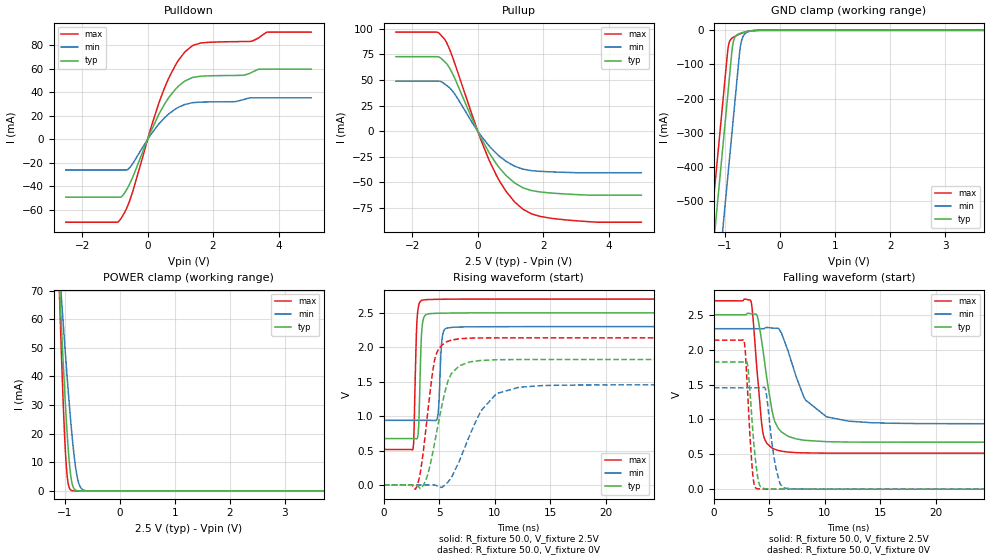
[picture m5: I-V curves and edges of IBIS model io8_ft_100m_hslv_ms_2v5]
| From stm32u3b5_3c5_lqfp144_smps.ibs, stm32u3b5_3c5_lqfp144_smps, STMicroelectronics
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[Model]   io8_ft_100m_hslv_ms_2v5
Model_type I/O
Polarity   Non-Inverting
Enable   Active-Low
| CAP_THRESHOLD on pad IOFT is "UDTCAPC" :
| Rising=30.0% of vddiom   Falling=70.0% of vddiom
| C_comp min and max val. don't necessarily correlate with the min and max pvt
| but are the smallest and greatest pad capacitance found.
| var   typ   min   max
C_comp   3.68195pF  3.67098pF  3.72549pF
|C_comp_pullup   2.08701pF  2.19344pF  2.32528pF
|C_comp_pulldown   1.59494pF  1.47754pF  1.40021pF
Vinl = 1.15V
Vinh = 1.35V
Vmeas = 1.25V   | Reference voltage for timing measurements
Cref  = 50.0pF   | Timing specification test load capacitance value
Rref  = 1.0MOhm   | Timing specification test load resistance value
Vref  = 1.375V   | Timing specification test load voltage
[Model Spec]
| TIME_THRESHOLD on pin ZIV11 is "CMOS" :
| Rising=50.0% of vdd   Falling=50.0% of vdd
Vinl 981.50000mV 911.50000mV 1.04650V
Vinh 1.42350V 1.31650V 1.50350V
| variable   typ   min   max
[Temperature Range] 25.0 130.0 -40.0
| variable   typ   min   max
[Voltage Range] 2.5V 2.3V 2.7V
| variable   typ   min   max
[POWER Clamp Reference] 2.5V 2.3V 2.7V
| variable   typ   min   max
[GND Clamp Reference] 0V 0V 0V
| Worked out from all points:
|   slope of the pulldown table from 0 to 0.375 V, typ, clamps not added: 16.4 ohm
|   slope of the pullup table from 0 to 0.375 V, typ, clamps not added: 16.7 ohm
|   GND clamp passes 1 mA (typ) near -0.50 V on its own axis
|   POWER clamp passes 1 mA (typ) near -0.83 V on its own axis
|   rising waveform, R_fixture 50.0, V_fixture 2.5V: 20-80 % time 200ps typ, 221ps min, 204ps max; typ from 0.673 V to 2.5 V
|   falling waveform, R_fixture 50.0, V_fixture 2.5V: 20-80 % time 1.06ns typ, 2.21ns min, 676ps max; typ from 2.5 V to 0.673 V
|   rising waveform, R_fixture 50.0, V_fixture 0V: 20-80 % time 1.41ns typ, 2.59ns min, 952ps max; typ from 0 V to 1.82 V
|   falling waveform, R_fixture 50.0, V_fixture 0V: 20-80 % time 567ps typ, 730ps min, 465ps max; typ from 1.82 V to 0 V
[POWER Clamp]
-2.5V     736.6mA    513.9mA    1.064A
-1.1V     75.38mA    79.63mA    73.18mA
-1.09V    71.2mA     76.8mA     67.14mA
-1.08V    67.05mA    73.98mA    61.2mA
-1.06V    58.89mA    68.38mA    49.67mA
-1.02V    43.22mA    57.4mA     28.67mA
-980mV    28.81mA    46.77mA    12.28mA
-940mV    16.45mA    36.61mA    3.257mA
-880mV    4.35mA     22.67mA    225.4uA
-770mV    97.5uA     4.87mA     1.193uA
-630mV    518.5nA    149.1uA    1.636nA
5V        0A         0A         0A
[GND Clamp]
-2.5V     -2.831A    -3.071A    -2.699A
-1.46V    -1.063A    -1.303A    -931.1mA
-1.21V    -637.8mA   -878.3mA   -506.1mA
-950mV    -195.8mA   -436.3mA   -64.07mA
-940mV    -178.8mA   -419.3mA   -50.67mA
-910mV    -127.8mA   -368.3mA   -31.36mA
-850mV    -37.25mA   -266.3mA   -20.72mA
-750mV    -10.68mA   -96.33mA   -12.3mA
-710mV    -8.126mA   -41.01mA   -9.515mA
-670mV    -6.142mA   -18.5mA    -7.051mA
-470mV    -612.4uA   -1.154mA   -431uA
5V        1.687nA    211.8nA    737.8pA
| variable   typ   min   max
[Pullup Reference] 2.5V 2.3V 2.7V
| variable   typ   min   max
[Pulldown Reference] 0V 0V 0V
[Pullup]
-2.5V     72.7mA     48.83mA    96.68mA
-1.25V    72.7mA     48.83mA    96.66mA
-1.01V    67.66mA    46.06mA    89.69mA
-750mV    54.85mA    38.28mA    70.46mA
0V        571.7fA    142.4pA    3.43fA
350mV     -21.19mA   -14.53mA   -28.53mA
850mV     -42.77mA   -29.12mA   -58.03mA
1.13V     -50.64mA   -34.25mA   -69.19mA
1.38V     -55.27mA   -37.08mA   -76.15mA
1.9V      -59.33mA   -39.2mA    -83.14mA
2.5V      -60.98mA   -40.04mA   -86.01mA
5V        -62.43mA   -40.58mA   -88.86mA
[Pulldown]
-2.5V     -49.09mA   -26.02mA   -70.37mA
-920mV    -49.09mA   -26.02mA   -70.37mA
-830mV    -49.09mA   -26.02mA   -67.8mA
-510mV    -35.57mA   -22.69mA   -49.05mA
90mV      6.138mA    3.798mA    8.848mA
520mV     30.1mA     18.41mA    43.96mA
940mV     45.18mA    27.25mA    67.1mA
1.38V     52.7mA     31.24mA    79.88mA
2.68V     54.32mA    32.09mA    83.06mA
3.2V      57.2mA     35.33mA    83.52mA
3.67V     59.71mA    35.33mA    91.16mA
5V        59.71mA    35.33mA    91.17mA
[Ramp]
dV/dt_r 1.09344V/1.40251ns 871.77536mV/2.40316ns 1.28161V/950.66097ps
dV/dt_f 1.09609V/1.06397ns 816.98943mV/1.93326ns 1.31053V/675.62203ps
R_load = 50.0
| Removed startup time: 0s 0s 0s  .
| Removed end time: 34.25ns.
[Rising Waveform]
R_fixture   = 50.0
V_fixture   = 2.5V
V_fixture_min = 2.3V
V_fixture_max = 2.7V
0s        673.2mV    938.4mV    515.8mV
2.65ns    673.2mV    938.4mV    528.7mV
3ns       670.5mV    938.4mV    2.391V
3.15ns    840.3mV    938.4mV    2.605V
3.4ns     2.162V     938.4mV    2.679V
3.7ns     2.457V     938.4mV    2.689V
4.85ns    2.494V     981.8mV    2.696V
5.25ns    2.495V     2.115V     2.697V
5.65ns    2.496V     2.277V     2.698V
34.25ns   2.5V       2.3V       2.7V
| Removed startup time: 0s 0s 0s  .
| Removed end time: 99.25ns.
[Falling Waveform]
R_fixture   = 50.0
V_fixture   = 2.5V
V_fixture_min = 2.3V
V_fixture_max = 2.7V
0s        2.5V       2.3V       2.7V
3.35ns    2.515V     2.3V       2.694V
3.9ns     2.488V     2.3V       1.686V
4.45ns    1.968V     2.299V     789.2mV
5.35ns    1.048V     2.309V     581.9mV
6.1ns     818.7mV    2.235V     544.4mV
8.25ns    699.3mV    1.279V     519.8mV
10.15ns   680.6mV    1.037V     516.6mV
12.15ns   675.3mV    974.7mV    516mV
99.25ns   673.2mV    938.4mV    515.8mV
| Removed startup time: 0s 0s 0s  .
| Removed end time: 99.2ns.
[Rising Waveform]
R_fixture   = 50.0
V_fixture   = 0V
V_fixture_min = 0V
V_fixture_max = 0V
0s        5.234nV    85.5nV     4.322nV
2.9ns     -1.384mV   -167.4nV   -49.07mV
3.35ns    -49.4mV    -3.978uV   229.8mV
3.85ns    93.87mV    -11.33uV   881.9mV
4.65ns    665.9mV    -2.479mV   1.854V
5.75ns    1.491V     35.77mV    2.084V
6.8ns     1.729V     341.6mV    2.123V
10.15ns   1.819V     1.326V     2.136V
14.2ns    1.822V     1.443V     2.136V
99.2ns    1.822V     1.453V     2.136V
| Removed startup time: 0s 0s 0s  .
| Removed end time: 34.2ns.
[Falling Waveform]
R_fixture   = 50.0
V_fixture   = 0V
V_fixture_min = 0V
V_fixture_max = 0V
0s        1.822V     1.453V     2.136V
2.7ns     1.823V     1.453V     2.143V
3.05ns    1.77V      1.453V     1.392V
3.45ns    968.2mV    1.453V     320.2mV
3.85ns    287.9mV    1.453V     9.804mV
4.15ns    50.73mV    1.453V     3.83mV
4.65ns    5.098mV    1.434V     2.244mV
5.5ns     2.174mV    382.7mV    1.365mV
6.3ns     1.489mV    18.25mV    805.6uV
34.2ns    50.87nV    781.9nV    14.06nV
